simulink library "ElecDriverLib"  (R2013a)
settings: Solver=ode45  StartTime=0.0  StopTime=10.0  RelTol=1e-3
undefined symbols (not defined in the file or in its folder): DriverParam, SimParam

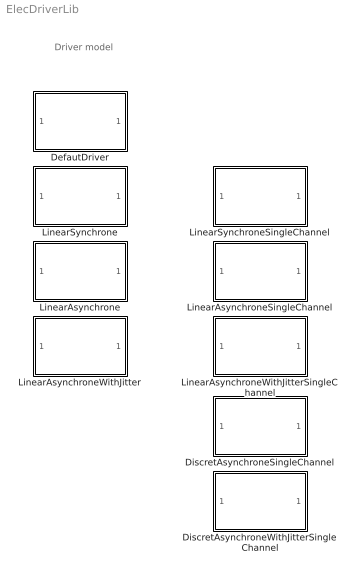
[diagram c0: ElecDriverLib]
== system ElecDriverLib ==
  note: Driver model
  DefautDriver : Subsystem  InitFcn=DriverParam = driver_ParamInitFnc(RawParam,1);  VariantControl=driverVarDefault
  DiscretAsynchroneSingleChannel : Subsystem  InitFcn=SimParam.Driver = driver_ParamInitFnc(RawParam,4);  VariantControl=driverVarLinearAsynchroneWithJitter
  DiscretAsynchroneWithJitterSingleChannel : Subsystem  InitFcn=SimParam.Driver = driver_ParamInitFnc(RawParam,4);  VariantControl=driverVarLinearAsynchroneWithJitter
  LinearAsynchrone : Subsystem  InitFcn=SimParam.Driver = driver_ParamInitFnc(RawParam,3);  VariantControl=driverVarLinearAsynchrone
  LinearAsynchroneSingleChannel : Subsystem  InitFcn=SimParam.Driver = driver_ParamInitFnc(RawParam,3);  VariantControl=driverVarLinearAsynchroneWithJitter
  LinearAsynchroneWithJitter : Subsystem  InitFcn=SimParam.Driver = driver_ParamInitFnc(RawParam,3);  VariantControl=driverVarLinearAsynchroneWithJitter
  LinearAsynchroneWithJitterSingleChannel : Subsystem  InitFcn=SimParam.Driver = driver_ParamInitFnc(RawParam,3);  VariantControl=driverVarLinearAsynchroneWithJitter
  LinearSynchrone : Subsystem  InitFcn=DriverParam = driver_ParamInitFnc(RawParam,2);  VariantControl=driverVarLinearSynchrone
  LinearSynchroneSingleChannel : Subsystem  InitFcn=SimParam.Driver = driver_ParamInitFnc(RawParam,2);  VariantControl=driverVarLinearSynchrone

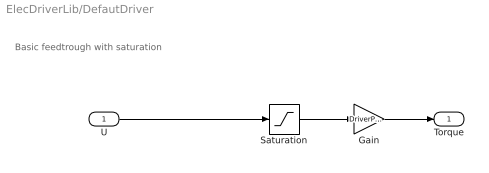
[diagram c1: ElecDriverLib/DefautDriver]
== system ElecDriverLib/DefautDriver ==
  note: Basic feedtrough with saturation
  U : Inport
  Gain : Gain  Gain=DriverParam.GRelScale
  Saturation : Saturate  UpperLimit=DriverParam.Sat  LowerLimit=-DriverParam.Sat
  Torque : Outport
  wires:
  U/1 -> Saturation/1
  Saturation/1 -> Gain/1
  Gain/1 -> Torque/1

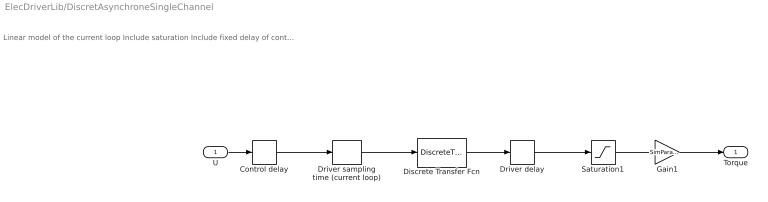
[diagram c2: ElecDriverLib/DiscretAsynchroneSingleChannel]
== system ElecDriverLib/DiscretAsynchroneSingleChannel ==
  note: Linear model of the current loop Include saturation Include fixed delay of control and driver and sampling time
  U : Inport
  Control delay : TransportDelay  DelayTime=SimParam.Driver.tau1
  Discrete Transfer Fcn : DiscreteTransferFcn  Numerator=SimParam.Driver.TfNum  Denominator=SimParam.Driver.TfDen
  Driver delay : TransportDelay  DelayTime=SimParam.Driver.tau2
  Driver sampling time (current loop) : ZeroOrderHold  SampleTime=SimParam.Driver.Te
  Gain1 : Gain  Gain=SimParam.Driver.GRelScale
  Saturation1 : Saturate  UpperLimit=SimParam.Driver.Sat  LowerLimit=-SimParam.Driver.Sat
  Torque : Outport
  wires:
  Gain1/1 -> Torque/1
  Saturation1/1 -> Gain1/1
  Discrete Transfer Fcn/1 -> Driver delay/1
  U/1 -> Control delay/1
  Driver delay/1 -> Saturation1/1
  Control delay/1 -> Driver sampling time (current loop)/1
  Driver sampling time (current loop)/1 -> Discrete Transfer Fcn/1

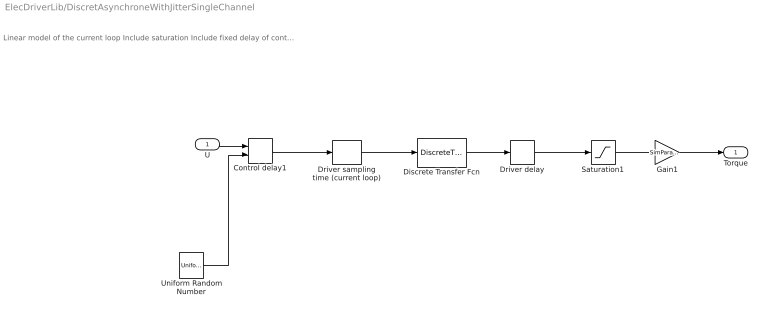
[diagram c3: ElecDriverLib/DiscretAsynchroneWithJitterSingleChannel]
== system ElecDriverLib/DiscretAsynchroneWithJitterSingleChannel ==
  note: Linear model of the current loop Include saturation Include fixed delay of control and driver and sampling time
  U : Inport
  Control delay1 : VariableTransportDelay  VariableDelayType=Variable transport delay  MaximumDelay=SimParam.Driver.tau1*2
  Discrete Transfer Fcn : DiscreteTransferFcn  Numerator=SimParam.Driver.TfNum  Denominator=SimParam.Driver.TfDen
  Driver delay : TransportDelay  DelayTime=SimParam.Driver.tau2
  Driver sampling time (current loop) : ZeroOrderHold  SampleTime=SimParam.Driver.Te
  Gain1 : Gain  Gain=SimParam.Driver.GRelScale
  Saturation1 : Saturate  UpperLimit=SimParam.Driver.Sat  LowerLimit=-SimParam.Driver.Sat
  Uniform Random Number : UniformRandomNumber  Minimum=SimParam.Driver.tau1*0.95  Maximum=SimParam.Driver.tau1*1.05  SampleTime=SimParam.Driver.TeControl
  Torque : Outport
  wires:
  Gain1/1 -> Torque/1
  Saturation1/1 -> Gain1/1
  Discrete Transfer Fcn/1 -> Driver delay/1
  U/1 -> Control delay1/1
  Driver delay/1 -> Saturation1/1
  Control delay1/1 -> Driver sampling time (current loop)/1
  Driver sampling time (current loop)/1 -> Discrete Transfer Fcn/1
  Uniform Random Number/1 -> Control delay1/2

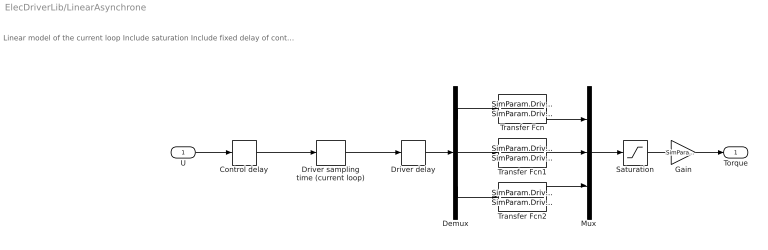
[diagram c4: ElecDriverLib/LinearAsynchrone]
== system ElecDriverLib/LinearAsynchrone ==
  note: Linear model of the current loop Include saturation Include fixed delay of control and driver and sampling time
  U : Inport
  Control delay : TransportDelay  DelayTime=SimParam.Driver.tau1
  Demux : Demux  Outputs=3
  Driver delay : TransportDelay  DelayTime=SimParam.Driver.tau2
  Driver sampling time (current loop) : ZeroOrderHold  SampleTime=SimParam.Driver.Te
  Gain : Gain  Gain=SimParam.Driver.GRelScale
  Mux : Mux  Inputs=3
  Saturation : Saturate  UpperLimit=SimParam.Driver.Sat  LowerLimit=-SimParam.Driver.Sat
  Transfer Fcn : TransferFcn  Numerator=SimParam.Driver.TfNum  Denominator=SimParam.Driver.TfDen
  Transfer Fcn1 : TransferFcn  Numerator=SimParam.Driver.TfNum  Denominator=SimParam.Driver.TfDen
  Transfer Fcn2 : TransferFcn  Numerator=SimParam.Driver.TfNum  Denominator=SimParam.Driver.TfDen
  Torque : Outport
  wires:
  U/1 -> Control delay/1
  Demux/1 -> Transfer Fcn/1
  Transfer Fcn/1 -> Mux/1
  Demux/3 -> Transfer Fcn2/1
  Transfer Fcn2/1 -> Mux/3
  Transfer Fcn1/1 -> Mux/2
  Demux/2 -> Transfer Fcn1/1
  Mux/1 -> Saturation/1
  Driver delay/1 -> Demux/1
  Control delay/1 -> Driver sampling time (current loop)/1
  Driver sampling time (current loop)/1 -> Driver delay/1
  Saturation/1 -> Gain/1
  Gain/1 -> Torque/1

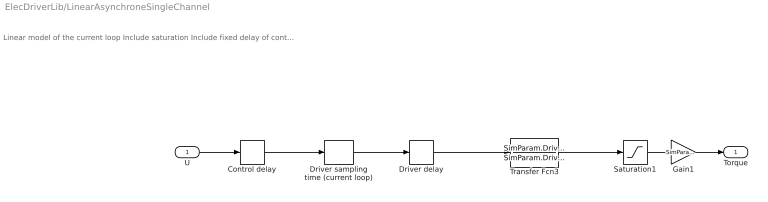
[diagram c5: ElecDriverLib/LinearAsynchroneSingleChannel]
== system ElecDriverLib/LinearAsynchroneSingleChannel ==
  note: Linear model of the current loop Include saturation Include fixed delay of control and driver and sampling time
  U : Inport
  Control delay : TransportDelay  DelayTime=SimParam.Driver.tau1
  Driver delay : TransportDelay  DelayTime=SimParam.Driver.tau2
  Driver sampling time (current loop) : ZeroOrderHold  SampleTime=SimParam.Driver.Te
  Gain1 : Gain  Gain=SimParam.Driver.GRelScale
  Saturation1 : Saturate  UpperLimit=SimParam.Driver.Sat  LowerLimit=-SimParam.Driver.Sat
  Transfer Fcn3 : TransferFcn  Numerator=SimParam.Driver.TfNum  Denominator=SimParam.Driver.TfDen
  Torque : Outport
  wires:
  U/1 -> Control delay/1
  Gain1/1 -> Torque/1
  Driver delay/1 -> Transfer Fcn3/1
  Saturation1/1 -> Gain1/1
  Transfer Fcn3/1 -> Saturation1/1
  Control delay/1 -> Driver sampling time (current loop)/1
  Driver sampling time (current loop)/1 -> Driver delay/1

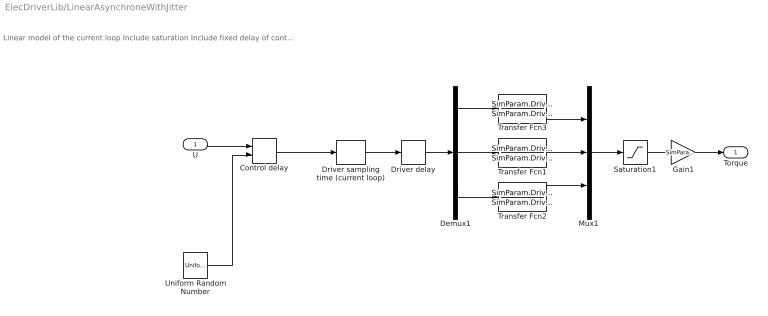
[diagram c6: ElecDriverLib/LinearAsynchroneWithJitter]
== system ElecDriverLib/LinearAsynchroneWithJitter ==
  note: Linear model of the current loop Include saturation Include fixed delay of control and driver and sampling time
  U : Inport
  Control delay : VariableTransportDelay  VariableDelayType=Variable transport delay  MaximumDelay=SimParam.Driver.tau1*2
  Demux1 : Demux  Outputs=3
  Driver delay : TransportDelay  DelayTime=SimParam.Driver.tau2
  Driver sampling time (current loop) : ZeroOrderHold  SampleTime=SimParam.Driver.Te
  Gain1 : Gain  Gain=SimParam.Driver.GRelScale
  Mux1 : Mux  Inputs=3
  Saturation1 : Saturate  UpperLimit=SimParam.Driver.Sat  LowerLimit=-SimParam.Driver.Sat
  Transfer Fcn1 : TransferFcn  Numerator=SimParam.Driver.TfNum  Denominator=SimParam.Driver.TfDen
  Transfer Fcn2 : TransferFcn  Numerator=SimParam.Driver.TfNum  Denominator=SimParam.Driver.TfDen
  Transfer Fcn3 : TransferFcn  Numerator=SimParam.Driver.TfNum  Denominator=SimParam.Driver.TfDen
  Uniform Random Number : UniformRandomNumber  Minimum=SimParam.Driver.tau1*0.99  Maximum=SimParam.Driver.tau1*1.01  SampleTime=SimParam.Driver.TeControl
  Torque : Outport
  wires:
  U/1 -> Control delay/1
  Control delay/1 -> Driver sampling time (current loop)/1
  Driver sampling time (current loop)/1 -> Driver delay/1
  Gain1/1 -> Torque/1
  Uniform Random Number/1 -> Control delay/2
  Demux1/1 -> Transfer Fcn3/1
  Transfer Fcn3/1 -> Mux1/1
  Demux1/3 -> Transfer Fcn2/1
  Transfer Fcn2/1 -> Mux1/3
  Transfer Fcn1/1 -> Mux1/2
  Demux1/2 -> Transfer Fcn1/1
  Mux1/1 -> Saturation1/1
  Driver delay/1 -> Demux1/1
  Saturation1/1 -> Gain1/1

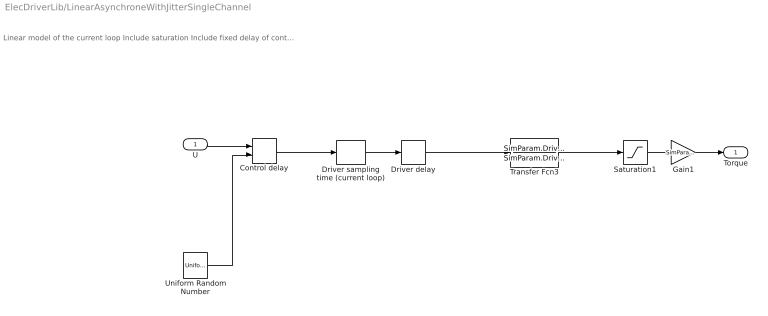
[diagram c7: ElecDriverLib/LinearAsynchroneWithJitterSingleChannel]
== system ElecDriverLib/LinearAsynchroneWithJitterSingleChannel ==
  note: Linear model of the current loop Include saturation Include fixed delay of control and driver and sampling time
  U : Inport
  Control delay : VariableTransportDelay  VariableDelayType=Variable transport delay  MaximumDelay=SimParam.Driver.tau1*2
  Driver delay : TransportDelay  DelayTime=SimParam.Driver.tau2
  Driver sampling time (current loop) : ZeroOrderHold  SampleTime=SimParam.Driver.Te
  Gain1 : Gain  Gain=SimParam.Driver.GRelScale
  Saturation1 : Saturate  UpperLimit=SimParam.Driver.Sat  LowerLimit=-SimParam.Driver.Sat
  Transfer Fcn3 : TransferFcn  Numerator=SimParam.Driver.TfNum  Denominator=SimParam.Driver.TfDen
  Uniform Random Number : UniformRandomNumber  Minimum=SimParam.Driver.tau1*0.99  Maximum=SimParam.Driver.tau1*1.01  SampleTime=SimParam.Driver.TeControl
  Torque : Outport
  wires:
  U/1 -> Control delay/1
  Control delay/1 -> Driver sampling time (current loop)/1
  Driver sampling time (current loop)/1 -> Driver delay/1
  Gain1/1 -> Torque/1
  Uniform Random Number/1 -> Control delay/2
  Driver delay/1 -> Transfer Fcn3/1
  Saturation1/1 -> Gain1/1
  Transfer Fcn3/1 -> Saturation1/1

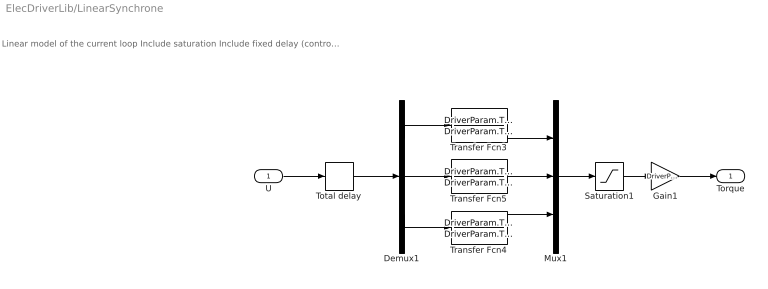
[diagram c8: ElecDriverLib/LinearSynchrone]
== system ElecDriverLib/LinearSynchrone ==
  note: Linear model of the current loop Include saturation Include fixed delay (control delay + driver delay + 0.5*driver sample periode if assynchonous)
  U : Inport
  Demux1 : Demux  Outputs=3
  Gain1 : Gain  Gain=DriverParam.GRelScale
  Mux1 : Mux  Inputs=3
  Saturation1 : Saturate  UpperLimit=DriverParam.Sat  LowerLimit=-DriverParam.Sat
  Total delay : TransportDelay  DelayTime=DriverParam.tau
  Transfer Fcn3 : TransferFcn  Numerator=DriverParam.TfNum  Denominator=DriverParam.TfDen
  Transfer Fcn4 : TransferFcn  Numerator=DriverParam.TfNum  Denominator=DriverParam.TfDen
  Transfer Fcn5 : TransferFcn  Numerator=DriverParam.TfNum  Denominator=DriverParam.TfDen
  Torque : Outport
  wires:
  U/1 -> Total delay/1
  Gain1/1 -> Torque/1
  Demux1/1 -> Transfer Fcn3/1
  Transfer Fcn3/1 -> Mux1/1
  Demux1/3 -> Transfer Fcn4/1
  Transfer Fcn4/1 -> Mux1/3
  Transfer Fcn5/1 -> Mux1/2
  Demux1/2 -> Transfer Fcn5/1
  Mux1/1 -> Saturation1/1
  Total delay/1 -> Demux1/1
  Saturation1/1 -> Gain1/1

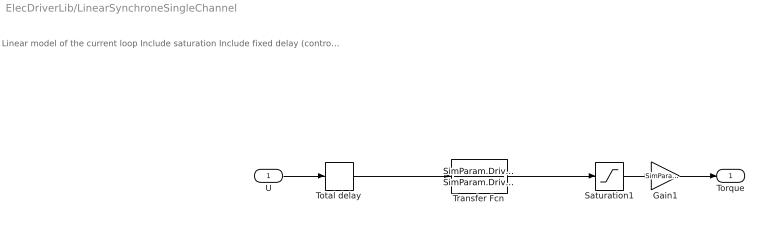
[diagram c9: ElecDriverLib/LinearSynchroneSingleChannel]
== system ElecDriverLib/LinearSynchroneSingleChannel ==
  note: Linear model of the current loop Include saturation Include fixed delay (control delay + driver delay + 0.5*driver sample periode if assynchonous)
  U : Inport
  Gain1 : Gain  Gain=SimParam.Driver.GRelScale
  Saturation1 : Saturate  UpperLimit=SimParam.Driver.Sat  LowerLimit=-SimParam.Driver.Sat
  Total delay : TransportDelay  DelayTime=SimParam.Driver.tau
  Transfer Fcn : TransferFcn  Numerator=SimParam.Driver.TfNum  Denominator=SimParam.Driver.TfDen
  Torque : Outport
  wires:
  U/1 -> Total delay/1
  Gain1/1 -> Torque/1
  Saturation1/1 -> Gain1/1
  Total delay/1 -> Transfer Fcn/1
  Transfer Fcn/1 -> Saturation1/1
